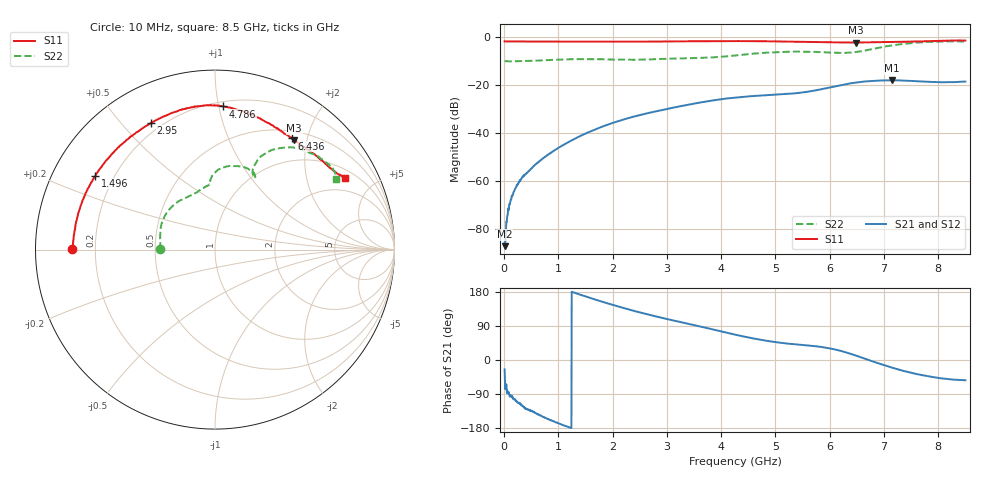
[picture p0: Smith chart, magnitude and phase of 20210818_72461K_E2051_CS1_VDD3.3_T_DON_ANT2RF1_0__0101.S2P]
!Agilent Technologies,E5071C,MY46417908,A.11.23
!Date: Wed Aug 18 14:24:10 2021
!Data & Calibration Information:
!Freq	S11:SOLT2(ON)	S21:SOLT2(ON)	S12:SOLT2(ON)	S22:SOLT2(ON)
!PortZ  Port1:50+j0  Port2:50+j0
!Above PortZ is port z conversion or system Z0 setting when saving the data.
!When reading, reference impedance value at option line is always used.
# Hz S dB R 50
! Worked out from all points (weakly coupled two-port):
!   1601 points, 10 MHz to 8.5 GHz, reference 50 ohm
!   highest |S21| = -18.19 dB at 7.152 GHz (marker M1); lowest = -87.2 dB at 15.31 MHz (marker M2)
!   lowest |S11| = -2.5 dB at 6.489 GHz (marker M3), VSWR 7.03, Z = 32 + j89.1 ohm
!   |S11| at or under -10 dB: nowhere
!   |S22| runs from -10.3 to -2.0 dB; largest |S21 - S12| = 0.00054
!   S11 on the Smith chart (normalised r, x): 10 MHz: 0.11, +0.00; 1.496 GHz: 0.13, +0.28; 2.95 GHz: 0.16, +0.60; 4.786 GHz: 0.23, +1.03; 6.436 GHz: 0.61, +1.74; 8.5 GHz: 1.33, +3.37
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1e7  -1.99 179.7  -85.82 -24.8  -90.07 -103.1  -10.26 179.6
1.530625e7  -2.01 179.6  -87.22 -53.9  -83.37 -73.7  -10.27 179.6
5.245e7  -2.03 178.9  -76.51 -86.8  -77.20 -82.8  -10.28 178.7
1.002062e8  -2.03 177.9  -69.75 -93.7  -69.71 -93.5  -10.29 177.5
1.426562e8  -2.03 177.0  -66.23 -98.3  -66.60 -97.1  -10.30 176.4
2.328625e8  -2.05 175.0  -61.90 -109.8  -62.19 -108.3  -10.28 174.1
3.336812e8  -2.04 173.0  -58.50 -121.0  -58.62 -120.8  -10.22 172.1
7.741e8  -2.08 163.6  -49.73 -153.7  -49.71 -154.1  -9.82 160.3
1.426769e9  -2.11 149.8  -41.13 171.3  -41.15 171.4  -9.40 139.2
1.49575e9  -2.11 148.3  -40.42 168.1  -40.42 168.1  -9.40 136.9
2.137806e9  -2.12 134.2  -34.95 139.9  -34.97 140.0  -9.61 118.2
2.843538e9  -2.06 119.0  -30.88 113.5  -30.88 113.5  -9.36 105.0
2.949662e9  -2.05 116.8  -30.35 109.8  -30.35 109.9  -9.28 103.4
4.255e9  -1.89 94.4  -25.38 67.1  -25.38 67.1  -7.89 92.7
4.785625e9  -1.95 86.7  -24.46 51.9  -24.46 52.0  -6.78 84.5
5.671769e9  -2.24 71.3  -22.66 37.5  -22.67 37.7  -6.34 65.0
6.435869e9  -2.47 55.4  -19.29 14.0  -19.31 13.9  -6.53 63.5
6.488931e9  -2.49 54.0  -19.12 11.4  -19.15 11.3  -6.42 64.0
7.088538e9  -2.27 42.4  -18.21 -17.6  -18.24 -17.7  -3.89 60.3
7.152212e9  -2.24 41.2  -18.19 -20.3  -18.22 -20.3  -3.66 59.0
7.937538e9  -1.81 30.8  -18.91 -46.0  -18.89 -46.0  -2.10 39.0
8.5e9  -1.66 29.1  -18.73 -53.4  -18.74 -53.6  -2.13 30.4
